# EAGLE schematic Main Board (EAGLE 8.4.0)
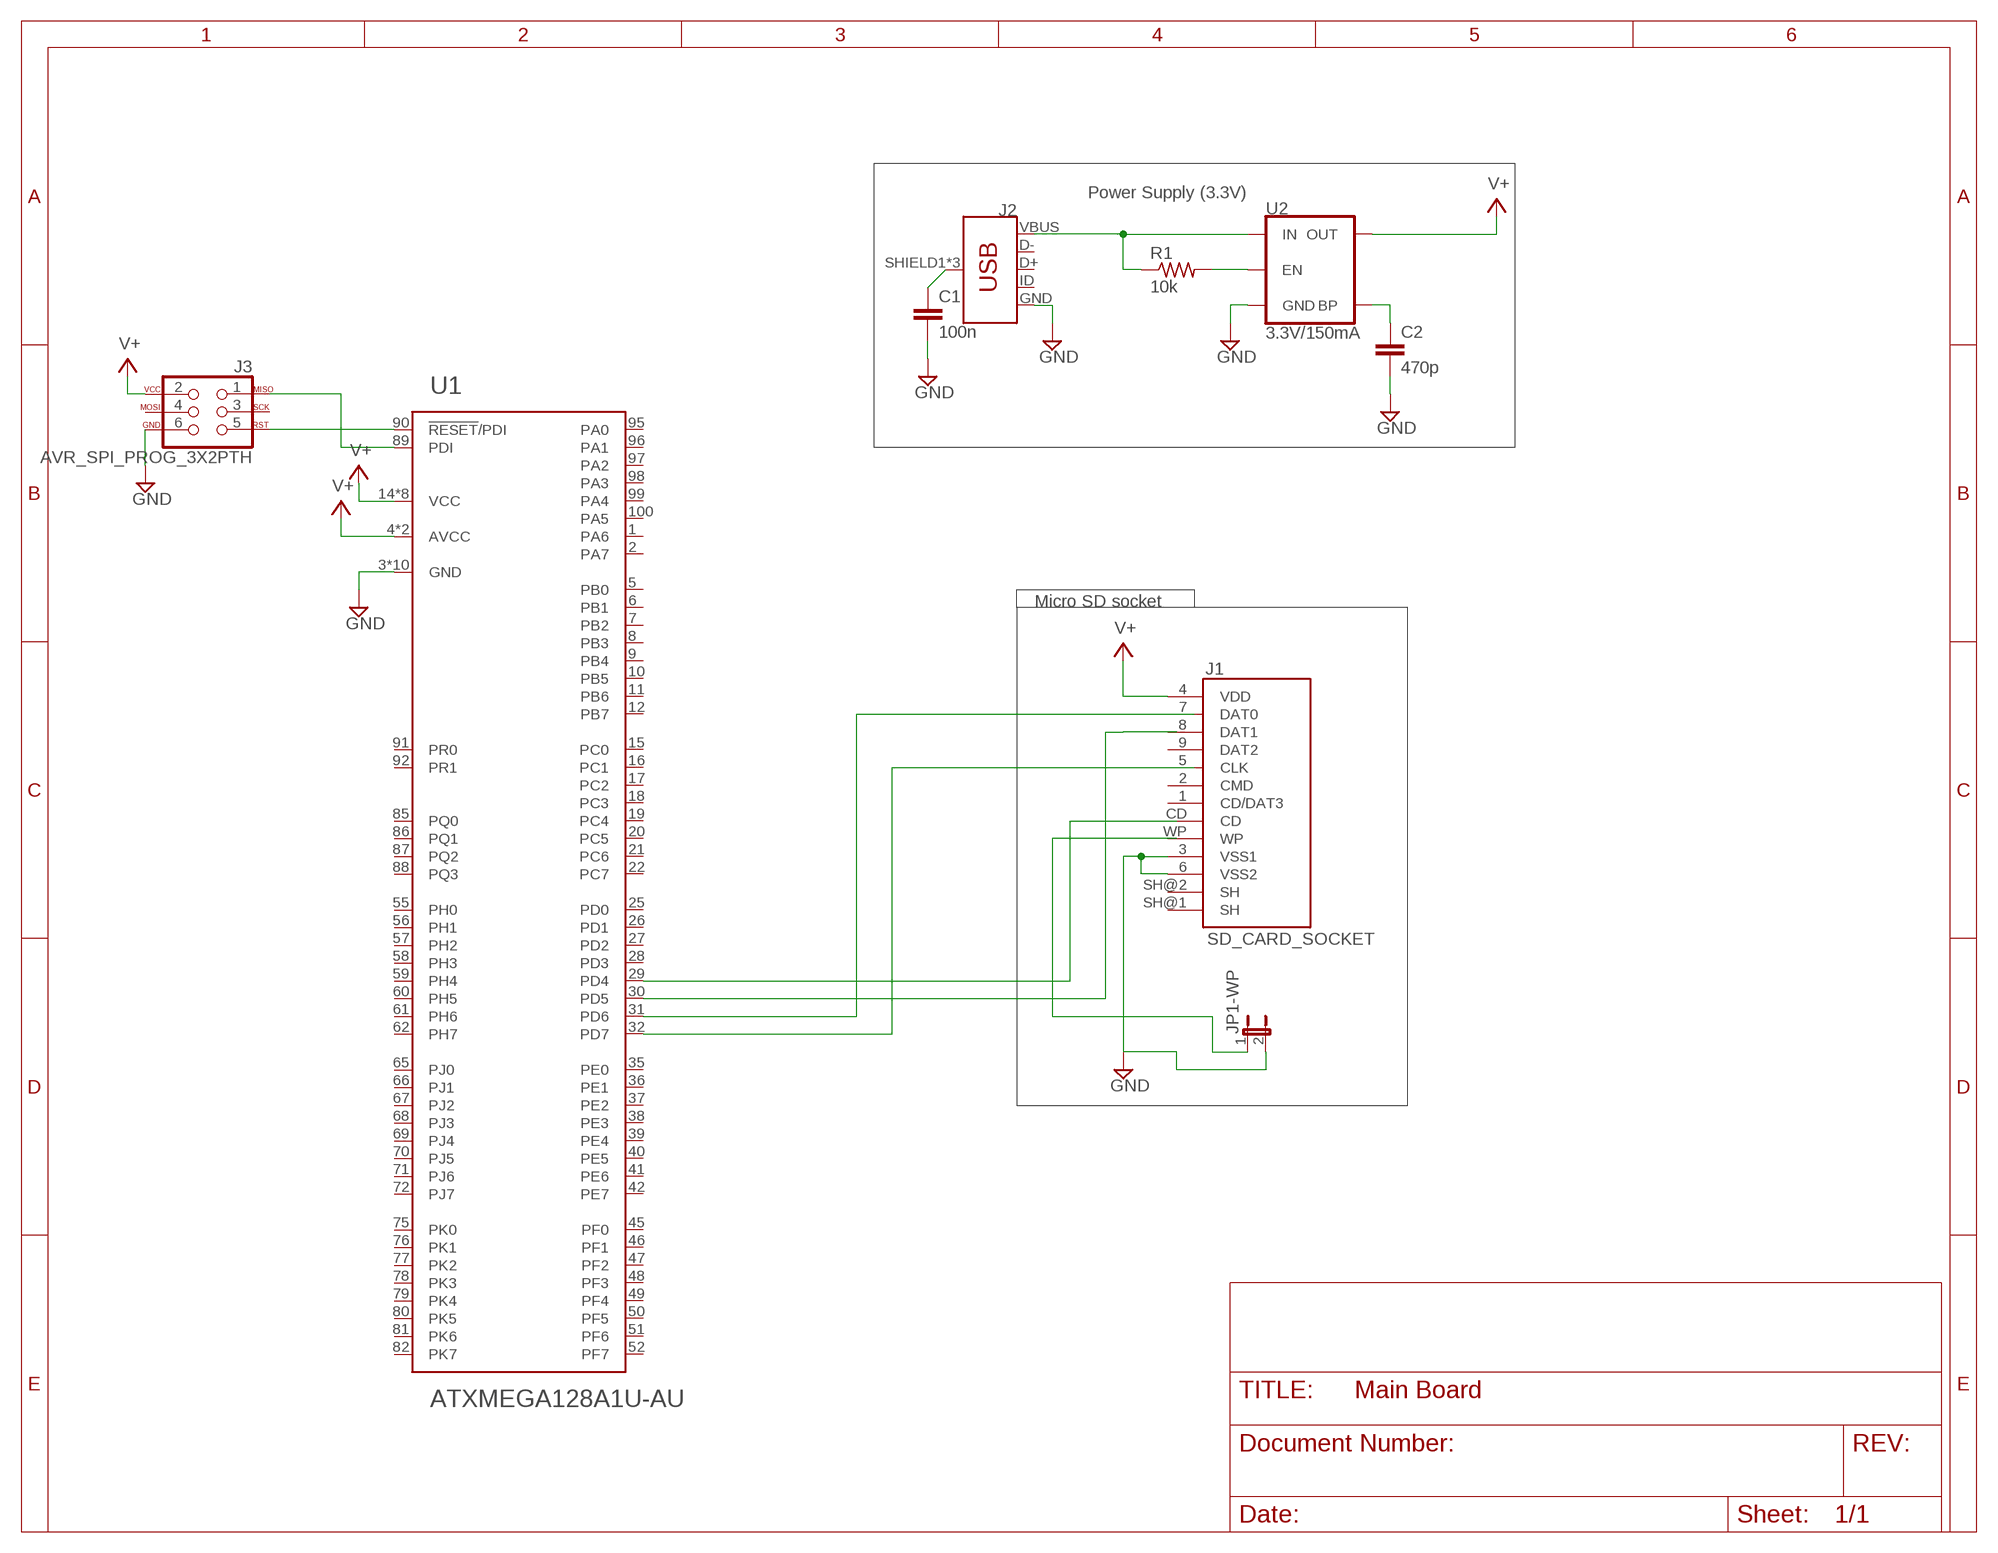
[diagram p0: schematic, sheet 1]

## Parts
C1  100n  C-EUC1206  [C1206]
C2  470p  C-EUC1206  [C1206]
J1  SD_CARD_SOCKET  [SD]
J2  USB_MICRO-B_FEMALE-SMT  [USB-B-MICRO-SMD]
J3  AVR_SPI_PROG_3X2PTH  [2X3]
JP1-WP  JUMPER-2PTH  [1X02]
R1  10k  R-US_M1206  [M1206]
U1  ATXMEGA128A1U-AU  [TQFP-100A-100]
U2  3.3V/150mA  V_REG_MIC52053.3V  [SOT23-5]

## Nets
BP: C2.1 U2.4(BP)
EN: R1.2 U2.3(EN)
GND: C1.2 C2.2 J1.3(VSS1) J1.6(VSS2) J2.GND J3.6 JP1-WP.2 U1.3(GND) U1.13(GND) U1.23(GND) U1.33(GND) U1.43(GND) U1.53(GND) U1.63(GND) U1.73(GND) U1.84(GND) U1.93(GND) U2.2(GND)
N$1: J3.5 U1.90(!RESET!/PDI)
N$2: J3.1 U1.89(PDI)
N$3: U1.31(PD6)
N$4: U1.32(PD7)
N$5: JP1-WP.1
N$7: U1.29(PD4)
N$8: U1.30(PD5)
SHIELD: C1.1 J2.SHIELD1(SHIELD) J2.SHIELD2(SHIELD) J2.SHIELD3(SHIELD)
V+: J1.4(VDD) J3.2 U1.4(AVCC) U1.14(VCC) U1.24(VCC) U1.34(VCC) U1.44(VCC) U1.54(VCC) U1.64(VCC) U1.74(VCC) U1.83(VCC) U1.94(AVCC) U2.5(OUT)
VIN: J2.VBUS R1.1 U2.1(IN)
Unconnected: J1.1(CD/DAT3) J1.2(CMD) J1.5(CLK) J1.7(DAT0) J1.8(DAT1) J1.9(DAT2) J1.CD J1.SH@1(SH) J1.SH@2(SH) J1.WP J2.D+ J2.D- J2.ID J3.3 J3.4 U1.1(PA6) U1.2(PA7) U1.5(PB0) U1.6(PB1) U1.7(PB2) U1.8(PB3) U1.9(PB4) U1.10(PB5) U1.11(PB6) U1.12(PB7) U1.15(PC0) U1.16(PC1) U1.17(PC2) U1.18(PC3) U1.19(PC4) U1.20(PC5) U1.21(PC6) U1.22(PC7) U1.25(PD0) U1.26(PD1) U1.27(PD2) U1.28(PD3) U1.35(PE0) U1.36(PE1) U1.37(PE2) U1.38(PE3) U1.39(PE4) U1.40(PE5) U1.41(PE6) U1.42(PE7) U1.45(PF0) U1.46(PF1) U1.47(PF2) U1.48(PF3) U1.49(PF4) U1.50(PF5) U1.51(PF6) U1.52(PF7) U1.55(PH0) U1.56(PH1) U1.57(PH2) U1.58(PH3) U1.59(PH4) U1.60(PH5) U1.61(PH6) U1.62(PH7) U1.65(PJ0) U1.66(PJ1) U1.67(PJ2) U1.68(PJ3) U1.69(PJ4) U1.70(PJ5) U1.71(PJ6) U1.72(PJ7) U1.75(PK0) U1.76(PK1) U1.77(PK2) U1.78(PK3) U1.79(PK4) U1.80(PK5) U1.81(PK6) U1.82(PK7) U1.85(PQ0) U1.86(PQ1) U1.87(PQ2) U1.88(PQ3) U1.91(PR0) U1.92(PR1) U1.95(PA0) U1.96(PA1) U1.97(PA2) U1.98(PA3) U1.99(PA4) U1.100(PA5)

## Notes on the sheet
- Power Supply (3.3V)
- Micro SD socket

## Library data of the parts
C1 C2 = rcl:C-EU: CAPACITOR, European symbol
J1 = SparkFun-Connectors:SD_CARD_SOCKET: SD Memory Card Connector (standard "large" size) Push-push normal type, CD enable, WP enable. Here is the connector we sell at SparkFun: SD/MMC Socket (PRT-12769) Datasheet It is used on these SparkFun products: SparkFun SD/MMC Card Breakout (BOB-12941) SD Sniffer (TOL-11468); PROD_ID: CONN-11976; SF_ID: PRT-12769
J2 = SparkFun-Connectors:USB_MICRO-B: USB Type Micro-B Connector Male/female and PTH/SMT variants SparkFun Products: SparkFun microB USB Breakout SparkFun USB microB Plug Breakout SparkFun ESP8266 Thing; PROD_ID: CONN-11752
J3 = SparkFun-Connectors:AVR_SPI_PROG_3X2: AVR ISP 6 Pin This is the reduced ISP connector for AVR programming. Common on Arduino. This footprint will take up less PCB space and can be used with a 10-pin to 6-pin adapter such as SKU: BOB-08508 **Special note about "TEST_POINT" package. The stop mask is on the top side, so if you want your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
JP1-WP = SparkFun-Retired:JUMPER-2: Jumper
R1 = rcl:R-US_: RESISTOR, American symbol
U1 = atmel-xmega:ATXMEGA128A1U: 8/16-bit XMEGA A1U Microcontroller Features High-performance, low-power Atmel® AVR® XMEGA® 8/16-bit Microcontroller Nonvolatileprogram and data memories – 64K - 128KBytes of in-system self-programmable flash – 4K - 8KBytes boot section – 2KBytes EEPROM – 4K - 8KBytes internal SRAM External bus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
U2 = SparkFun-IC-Power:V_REG_MIC5205: V_REG MIC5205 Standard 3.3V, 5V, and Adjustable 150mA LDO voltage regulator in SOT-23 layout. Micrel part MIC5205. BP (by-pass) pin is used to lower output noise with 470pF cap, may be left open. On the adjustable version BP is used to set output.; PROD_ID: VREG-00822

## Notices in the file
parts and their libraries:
SparkFun-IC-Power: Licensing: Creative Commons ShareAlike 4.0 International - https://creativecommons.org/licenses/by-sa/4.0
